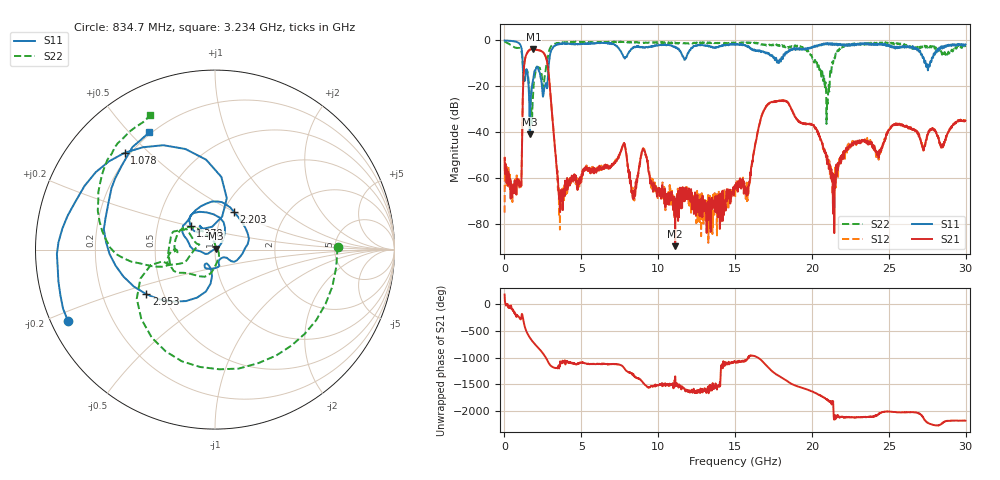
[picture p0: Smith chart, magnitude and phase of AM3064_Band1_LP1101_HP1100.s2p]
# Hz S DB R 50.0
!freq dBS11 angS11 dBS21 angS21 dBS12 angS12 dBS22 angS22
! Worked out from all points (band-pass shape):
!   1600 points, 10 MHz to 29.98 GHz, reference 50 ohm
!   highest |S21| = -3.75 dB at 1.884 GHz (marker M1); lowest = -89.8 dB at 11.11 GHz (marker M2)
!   |S21| within 3 dB of the highest: 1.393 GHz to 2.659 GHz (1.267 GHz wide, 62.5 % of centre)
!   lowest |S11| = -41.0 dB at 1.641 GHz (marker M3), VSWR 1.02, Z = 50.7 + j0.594 ohm
!   |S11| at or under -10 dB: 1.187 GHz to 2.891 GHz (1.705 GHz wide, 83.6 % of centre); 27.4 GHz to 27.68 GHz (281.5 MHz wide, 1.02 % of centre)
!   |S22| runs from -36.5 to -0.4 dB; largest |S21 - S12| = 0.011
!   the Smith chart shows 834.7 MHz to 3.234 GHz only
!   S11 on the Smith chart (normalised r, x): 834.7 MHz: 0.05, -0.23; 1.078 GHz: 0.18, +0.42; 1.378 GHz: 0.74, +0.20; 2.203 GHz: 1.12, +0.50; 2.953 GHz: 0.40, -0.25; 3.234 GHz: 0.19, +0.57
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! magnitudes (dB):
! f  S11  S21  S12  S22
! 10 MHz  0.0  -51.4  -75.1  -0.4
! 834.7 MHz  -0.8  -60.3  -63.3  -3.3
! 1.078 GHz  -2.6  -62.2  -63.3  -4.0
! 1.378 GHz  -14.5  -7.0  -7.0  -13.2
! 1.641 GHz  -41.0  -4.1  -4.1  -22.3
! 1.884 GHz  -16.4  -3.7  -3.8  -20.8
! 2.203 GHz  -12.6  -4.3  -4.2  -11.8
! 2.953 GHz  -6.8  -20.3  -20.3  -3.6
! 3.234 GHz  -2.5  -42.7  -43.0  -1.6
! 3.665 GHz  -1.6  -65.4  -65.4  -0.9
! 5.015 GHz  -1.6  -58.7  -58.6  -0.6
! 7.751 GHz  -7.2  -45.0  -45.2  -0.7
! 8.37 GHz  -3.1  -69.2  -67.6  -1.0
! 10 GHz  -2.1  -65.0  -66.5  -0.9
! 11.11 GHz  -3.1  -89.8  -77.2  -1.2
! 15 GHz  -1.8  -63.2  -68.3  -1.4
! 17.16 GHz  -5.6  -27.8  -27.6  -2.3
! 19.99 GHz  -3.3  -36.7  -36.8  -6.9
! 20.98 GHz  -1.3  -54.0  -51.4  -26.4
! 21.42 GHz  -1.6  -58.4  -61.5  -7.7
! 25 GHz  -1.9  -39.2  -38.9  -1.3
! 29.98 GHz  -1.8  -35.1  -35.0  -2.9
